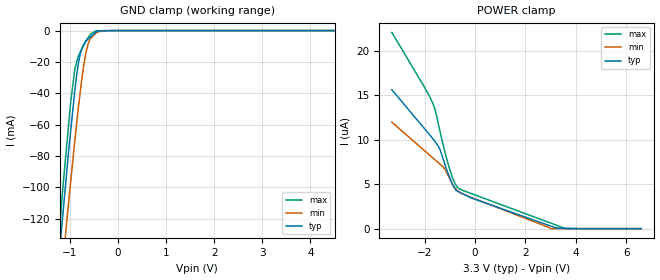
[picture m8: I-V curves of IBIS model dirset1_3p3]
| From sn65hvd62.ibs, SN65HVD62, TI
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|   dirset1_3p3 Model
[Model]   dirset1_3p3
Model_type   Input
Vinl = 0.99
Vinh = 2.3
|   typ   min   max
|   (nom PVT)   (fast PVT)   (slow PVT)
 C_comp   2.130e-12   2.058e-12   2.273e-12
| Where nom  PVT is Nominal Process, 3.3V, 27C
|   Fast PVT is Strong Process,  3.6V, -40C
|   Slow PVT is Weak Process,   3V, 125C
[Voltage Range]   3.3   3   3.6
|Ambient Temperature   25   85   -40
|Junction Temperature
[Temperature Range]   27   125   -40
[Power Clamp Reference]   3.3   3   3.6
[GND Clamp Reference]   0   0   0
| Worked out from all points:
|   GND clamp passes 1 mA (typ) near -0.46 V on its own axis
[GND Clamp]
|   Voltage   I(typ)   I(min)   I(max)
-3.3V     -947.8mA   -925.2mA   -980.3mA
-1.221V   -143.6mA   -173.4mA   -128.9mA
-1.127V   -111.7mA   -142.7mA   -94.47mA
-1.05V    -85.6mA    -117.7mA   -68.63mA
-986.4mV  -65.69mA   -98.16mA   -47.22mA
-896.4mV  -38.46mA   -70.48mA   -24.78mA
-815.1mV  -19.83mA   -47.53mA   -15.96mA
-745.8mV  -11.43mA   -30.06mA   -11.13mA
-654mV    -6.419mA   -12.56mA   -6.007mA
-570mV    -4.068mA   -5.034mA   -2.342mA
-450mV    -710.2uA   -1.366mA   -173.9uA
6.6V      0A         0A         0A
[POWER Clamp]
|   Voltage   I(typ)   I(min)   I(max)
-3.3V     15.61uA    11.96uA    22.04uA
-2.048V   11.38uA    8.876uA    16.11uA
-1.667V   10.08uA    7.936uA    14.04uA
-1.562V   9.685uA    7.678uA    13.14uA
-1.376V   8.804uA    7.219uA    10.8uA
-1.179V   7.081uA    6.618uA    8.471uA
-1.015V   5.831uA    5.691uA    6.777uA
-799.2mV  4.505uA    4.599uA    5.11uA
-622.8mV  4.11uA     4.106uA    4.474uA
3.003V    297.6nA    0A         628.1nA
3.596V    40.16nA    0A         0A
6.6V      0A         0A         0A
